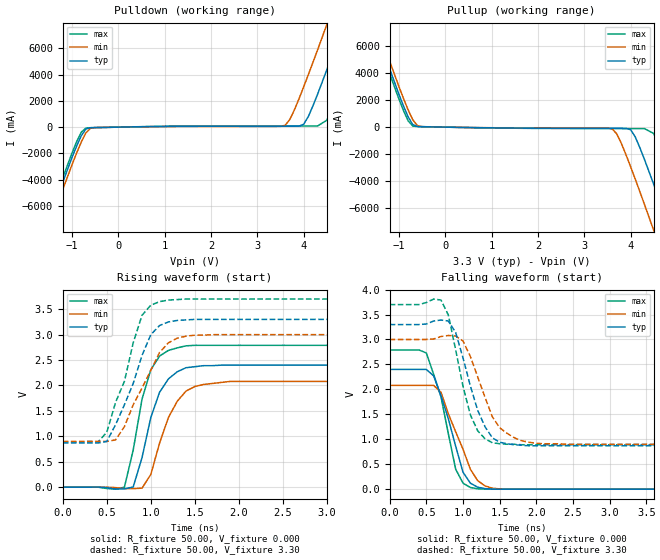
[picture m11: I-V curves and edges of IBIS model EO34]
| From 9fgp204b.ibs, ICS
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|   Model EO34
[Model]   EO34
Model_type   Output
Polarity   Non-Inverting
Vmeas =   1.50V
C_comp   3.40pF   2.85pF   3.95pF
[Temperature Range]   27.00   70.00   0.000
[Voltage Range]   3.30V   3.00V   3.70V
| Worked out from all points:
|   slope of the pulldown table from 0 to 0.495 V, typ, clamps not added: 15.9 ohm
|   slope of the pullup table from 0 to 0.495 V, typ, clamps not added: 17.1 ohm
|   rising waveform, R_fixture 50.00, V_fixture 0.000: 20-80 % time 237ps typ, 265ps min, 210ps max; typ from 0 V to 2.4 V
|   rising waveform, R_fixture 50.00, V_fixture 3.30: 20-80 % time 322ps typ, 350ps min, 292ps max; typ from 0.87 V to 3.3 V
|   falling waveform, R_fixture 50.00, V_fixture 0.000: 20-80 % time 286ps typ, 332ps min, 263ps max; typ from 2.4 V to 0 V
|   falling waveform, R_fixture 50.00, V_fixture 3.30: 20-80 % time 304ps typ, 340ps min, 262ps max; typ from 3.3 V to 0.87 V
[Pulldown]
| voltage   I(typ)   I(min)   I(max)
-3.3V     -24.68A    -25.4A     -24.36A
-1.7V     -8.95A     -9.49A     -8.61A
-1.5V     -7.01A     -7.56A     -6.67A
-900mV    -1.43A     -1.96A     -1.1A
-700mV    -140mA     -430mA     -67.64mA
3.6V      70.25mA    140mA      86.6mA
4V        220mA      3.07A      86.87mA
4.3V      2.51A      5.88A      87.78mA
4.5V      4.37A      7.81A      530mA
4.9V      8.22A      11.69A     4.03A
5.3V      12.13A     15.62A     7.88A
6.6V      24.98A     28.48A     20.69A
[Pullup]
| voltage   I(typ)   I(min)   I(max)
-3.3V     24.84A     25.38A     24.5A
-1.7V     9.1A       9.66A      8.75A
-1.5V     7.16A      7.73A      6.8A
-900mV    1.56A      2.12A      1.22A
-700mV    180mA      540mA      80.66mA
3.6V      -85.84mA   -120mA     -110mA
4V        -190mA     -2.93A     -110mA
4.3V      -2.4A      -5.74A     -110mA
4.5V      -4.25A     -7.67A     -470mA
4.9V      -8.1A      -11.56A    -3.93A
5.3V      -12.02A    -15.49A    -7.79A
6.6V      -24.9A     -28.38A    -20.62A
[Ramp]
| variable   typ   min   max
dV/dt_r   1.44/0.23n   1.25/0.26n   1.67/0.19n
dV/dt_f   1.46/0.29n   1.26/0.35n   1.68/0.25n
R_load = 50.00
[Rising Waveform]
R_fixture = 50.00
V_fixture = 0.000
V_fixture_min = 0.000
V_fixture_max = 0.000
| time   V(typ)   V(min)   V(max)
0s        0V         0V         0V
700ps     -33.34mV   -28.3mV    -1.14mV
800ps     4.88mV     -28.62mV   730mV
900ps     580mV      -18.71mV   1.73V
1ns       1.37V      250mV      2.31V
1.1ns     1.87V      870mV      2.58V
1.2ns     2.13V      1.37V      2.69V
1.4ns     2.35V      1.89V      2.78V
1.9ns     2.4V       2.08V      2.79V
5ns       2.4V       2.08V      2.79V
[Rising Waveform]
R_fixture = 50.00
V_fixture = 3.30
V_fixture_min = 3.00
V_fixture_max = 3.70
| time   V(typ)   V(min)   V(max)
0s        870mV      900mV      890mV
400ps     870mV      900mV      890mV
500ps     900mV      900mV      1.08V
600ps     1.23V      930mV      1.67V
700ps     1.62V      1.19V      2.08V
900ps     2.59V      1.95V      3.38V
1ns       3V         2.3V       3.58V
1.1ns     3.18V      2.65V      3.65V
1.5ns     3.3V       2.99V      3.7V
5ns       3.3V       3V         3.7V
[Falling Waveform]
R_fixture = 50.00
V_fixture = 0.000
V_fixture_min = 0.000
V_fixture_max = 0.000
| time   V(typ)   V(min)   V(max)
0s        2.4V       2.08V      2.79V
500ps     2.4V       2.08V      2.73V
600ps     2.27V      2.08V      2.3V
700ps     1.87V      1.94V      1.85V
900ps     860mV      1.15V      400mV
1ns       340mV      800mV      120mV
1.1ns     120mV      400mV      33.65mV
1.3ns     10.89mV    65.65mV    1.53mV
1.5ns     260uV      5.41mV     -38.56uV
5ns       -21.77uV   -20.38uV   -22.41uV
[Falling Waveform]
R_fixture = 50.00
V_fixture = 3.30
V_fixture_min = 3.00
V_fixture_max = 3.70
| time   V(typ)   V(min)   V(max)
0s        3.3V       3V         3.7V
700ps     3.39V      3.06V      3.79V
800ps     3.37V      3.08V      3.49V
900ps     3.14V      3.07V      2.79V
1.1ns     2.07V      2.66V      1.49V
1.2ns     1.58V      2.25V      1.17V
1.4ns     1.03V      1.45V      930mV
1.7ns     890mV      1.03V      900mV
2ns       870mV      920mV      890mV
5ns       870mV      900mV      890mV
